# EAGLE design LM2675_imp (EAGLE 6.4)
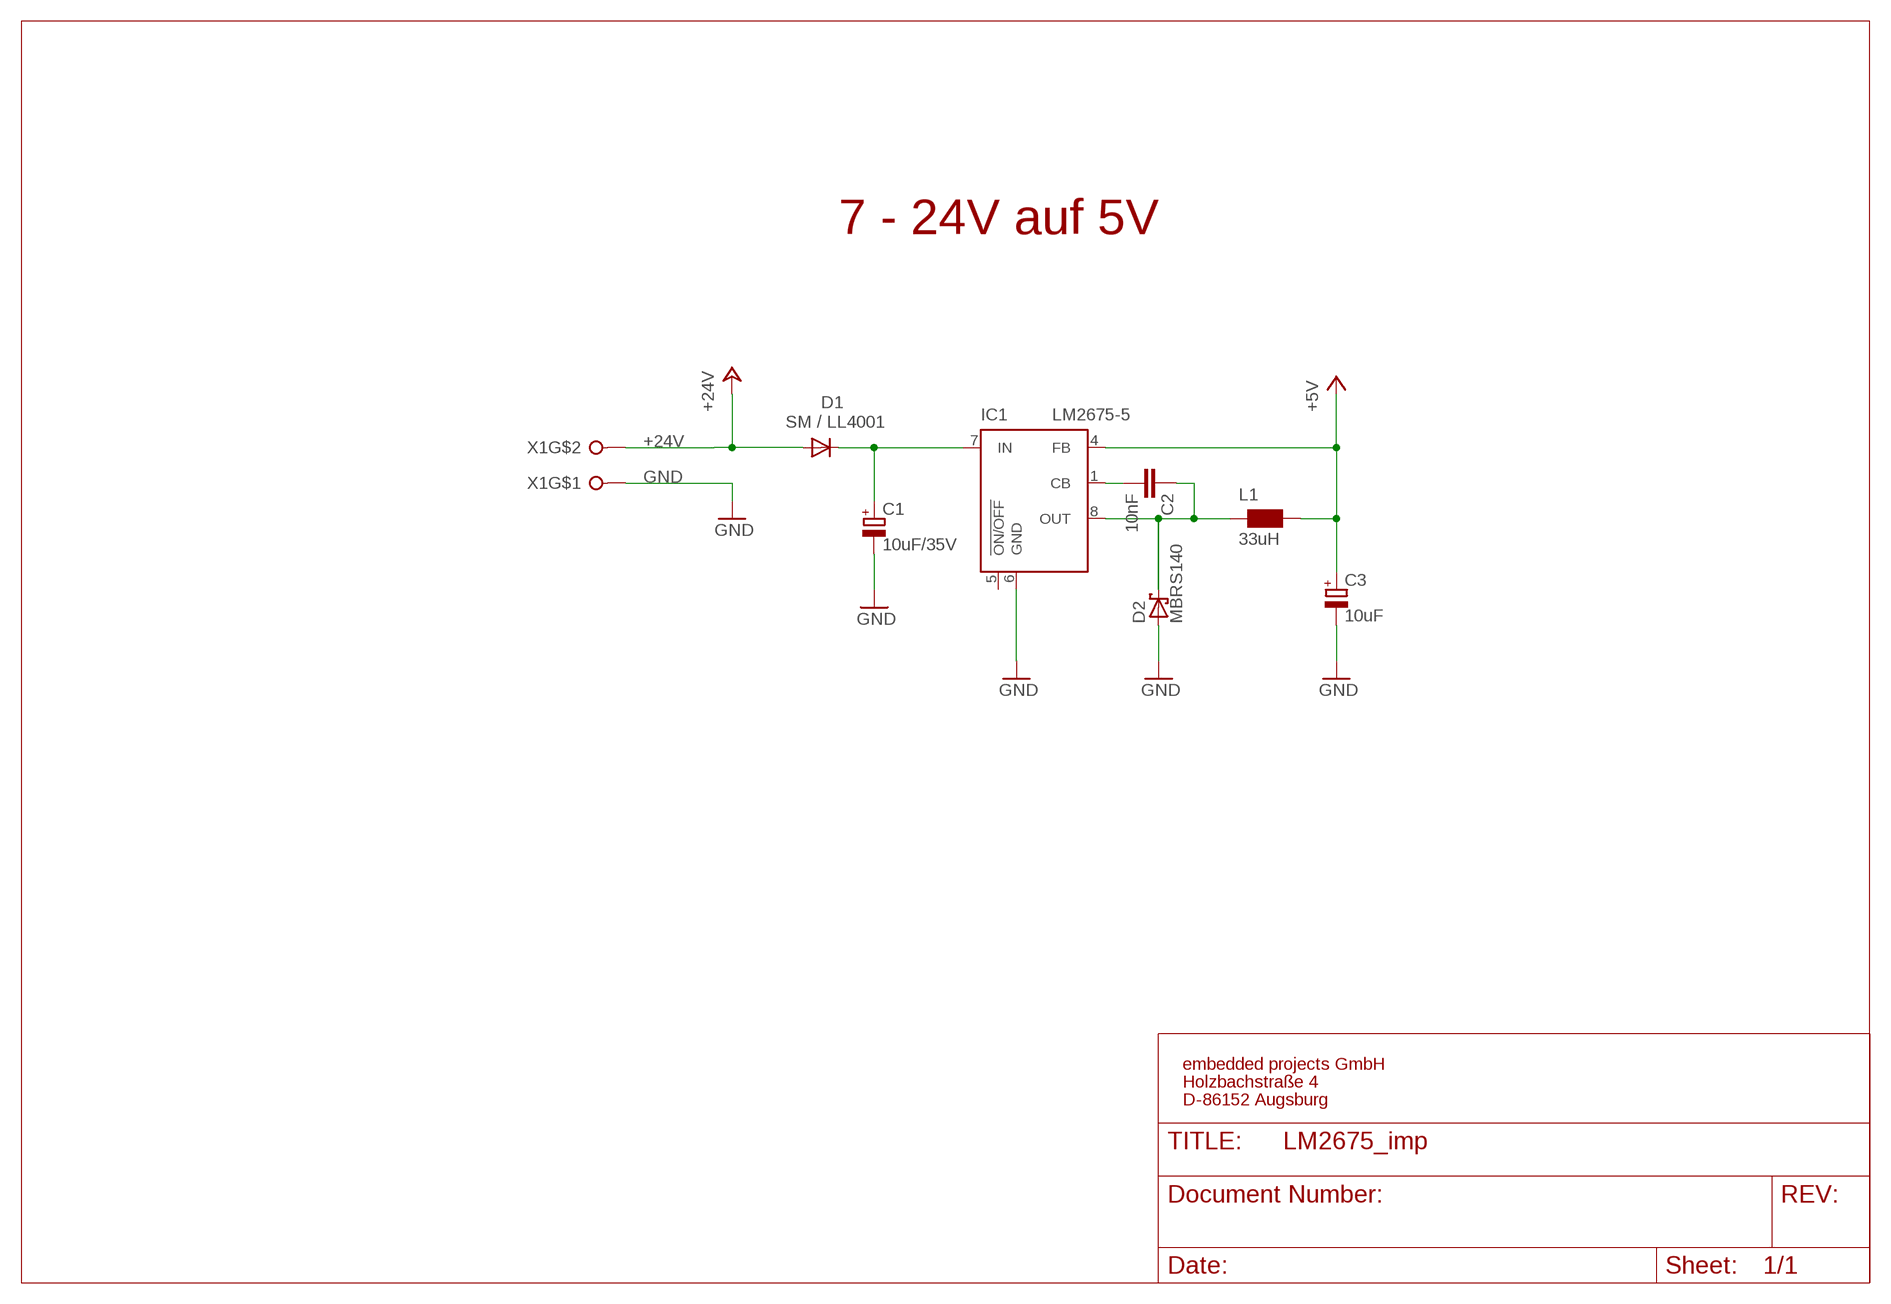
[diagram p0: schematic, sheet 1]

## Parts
C1  10uF/35V  CPOL-EUC  [PANASONIC_C]
C2  10nF  C-EUC0805  [C0805]
C3  10uF  CPOL-EUD/7343-31R  [D/7343-31R]
D1  SM / LL4001  DIODE-MINIMELF  [MINIMELF]
D2  MBRS140  MBRS130LT3  [SMB]
IC1  LM2675-5  LM2675MSO-8  [SO-8]
L1  33uH  WE-PD_S/M  [WE-PD_S/M]
X1  CON-WAGO508_W237-02  [W237-132]

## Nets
+5V: C3.+ IC1.4(FB) L1.1
+24V: D1.A X1.2
GND: C1.- C3.- D2.A IC1.6(GND) X1.1
N$40: C1.+ D1.C IC1.7(IN)
N$59: C2.2 IC1.1(CB)
OUT: C2.1 D2.C IC1.8(OUT) L1.2
Unconnected: IC1.5(!ON/OFF)

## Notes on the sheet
- 7 - 24V auf 5V
- embedded projects GmbH
- Holzbachstraße 4
- D-86152 Augsburg

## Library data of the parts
C1 = rcl:CPOL-EU: POLARIZED CAPACITOR, European symbol; EP: 400118; FARNELL: 9697012
C2 = rcl:C-EU: CAPACITOR, European symbol
C3 = rcl:CPOL-EU: POLARIZED CAPACITOR, European symbol
D1 = diode:DIODE-: DIODE; FARNELL: 7355521; POLLIN: 140697
D2 = diode:MBRS130LT3: Schottky Power Rectifier; EP: 400020
IC1 = LM2675M:LM2675M; EP: 400974; FARNELL: 9489746
L1 = Wurth_Electronics_Midcom_Speedy_and_standard_magnetics:WE-PD: SMD-Shielded Power Inductors WE-PD; EP: 400973; FARNELL: 744778133
X1 = EmbeddedProjectsBauteile:CON-WAGO508_W237-02: WAGO SREW CLAMP

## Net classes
0 default: width 0.2 mm, drill 0.3 mm, clearance 0.2 mm
1 500mA: width 0.3 mm, drill 0.3 mm, clearance 0.15 mm
2 5V: width 0.4 mm

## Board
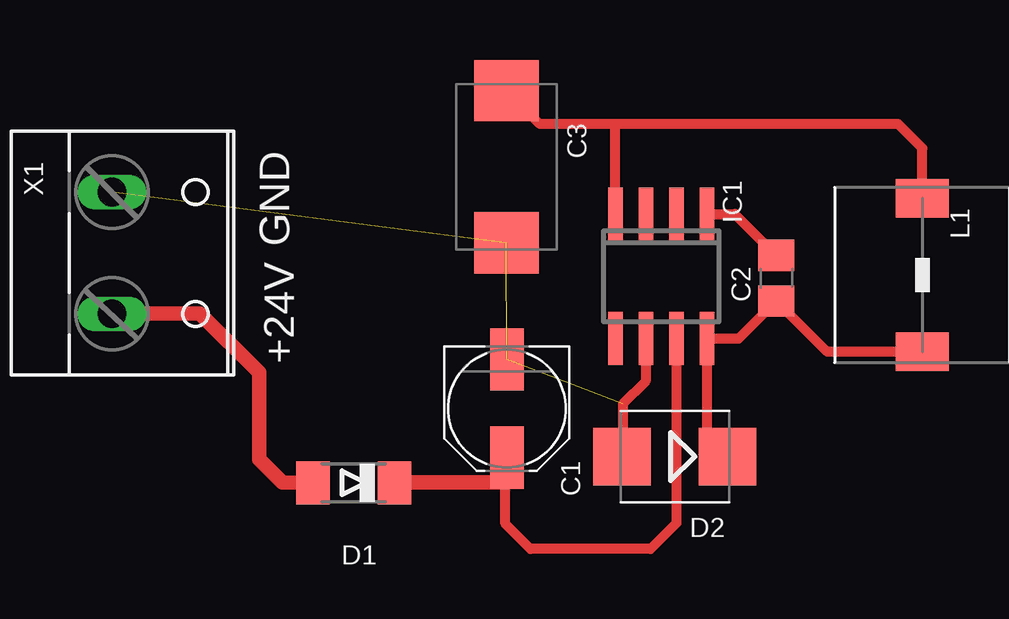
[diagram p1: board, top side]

No outline drawn. Coordinates in mm, seen from the top.
Copper layers (1*16): Top 0.012mm / dielectric 0.36mm / Bottom 0.012mm
Design rules "125um_0.2mmborhung_4Layer *": minimum track width 0.125mm, minimum drill 0.25mm, track to track 0.125mm, track to pad 0.125mm, pad to pad 0.125mm, via to via 0.125mm, smd to smd 0mil, copper to edge 0.4mm, drill to drill 0.3mm, minimum pad ring 0.125mm, minimum via ring 0.125mm, stop-mask expansion 0.125mm, vias tented up to drill 40mil, thermal gap 0.2mm

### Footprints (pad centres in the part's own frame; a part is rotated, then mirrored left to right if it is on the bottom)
PANASONIC_C = smd 2.6 x 1.4: + 2.05,0; - -2.05,0
C0805 = smd 1.3 x 1.5: 1 -0.95,0; 2 0.95,0
D/7343-31R = smd 2.55 x 2.7: + 3.175,0; - -3.175,0
MINIMELF = smd 1.4 x 1.8: A 1.7,0; C -1.7,0
SMB = smd 2.4 x 2.4: A 2.2,0; C -2.2,0
SO-8 = smd 0.6 x 2.2: 1 -1.905,-2.6; 2 -0.635,-2.6; 3 0.635,-2.6; 4 1.905,-2.6; 5 1.905,2.6; 6 0.635,2.6; 7 -0.635,2.6; 8 -1.905,2.6
WE-PD_S/M = smd 1.6 x 2.2: 1 -3.2,0; 2 3.2,0
W237-132 = drill 1.194 long: 1 -2.54,-0.635; 2 2.54,-0.635

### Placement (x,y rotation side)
C1  26.35,14.07 270 top
C2  37.58,19.51 90 top
C3  26.33,24.16 90 top
D1  19.97,10.98 180 top
D2  33.35,12.07 180 top
IC1  32.78,19.59 180 top
L1  43.66,19.64 270 top
X1  10.53,20.56 270 top

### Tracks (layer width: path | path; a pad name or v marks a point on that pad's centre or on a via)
+5V
  Top 0.406: L1.1 43.66,24.93 42.65,25.94 30.78,25.94 | 30.78,25.94 27.73,25.94 C3.+ | IC1.4 30.88,25.84 30.78,25.94
+24V
  Top 0.406: 9.9,18.03 X1.2
  Top 0.61: 9.9,18.03 12.97,18.03 13.56,18.03 16.03,15.57 16.03,11.96 17,11 D1.A
GND  (3 unrouted)
  Top 0.406: IC1.6 32.13,15.21 31.18,14.27 31.18,14.1 D2.A
N$40
  Top 0.254: 21.64,11.16 22.08,11
  Top 0.406: IC1.7 33.41,9.29 32.34,8.22 27.33,8.22 26.29,9.27 26.29,11.02 C1.+
  Top 0.61: D1.C 22.08,11 26.29,11 C1.+
N$59
  Top 0.406: IC1.1 35.85,22.19 C2.2
OUT
  Top 0.406: D2.C 34.69,13.15 IC1.8 36.01,16.99 C2.1 39.7,16.44 L1.2

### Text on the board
tPlace: GND | +24V

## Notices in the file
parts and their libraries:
Wurth_Electronics_Midcom_Speedy_and_stan: Copyright: Wurth Electronics Midcom, Inc.
